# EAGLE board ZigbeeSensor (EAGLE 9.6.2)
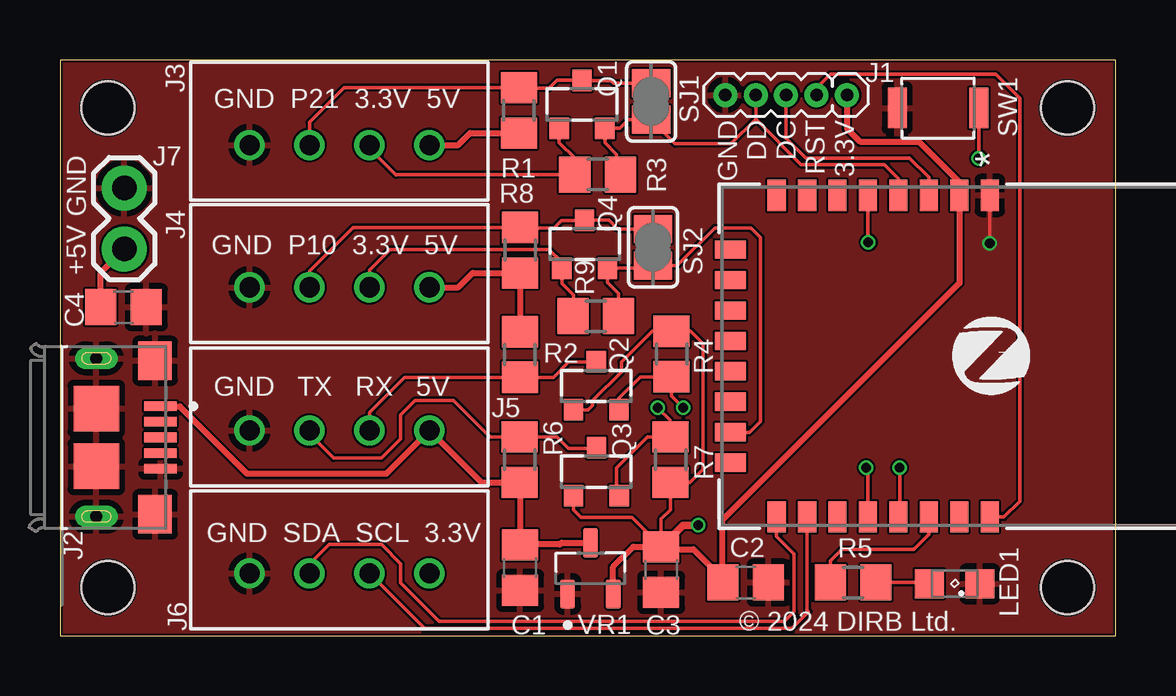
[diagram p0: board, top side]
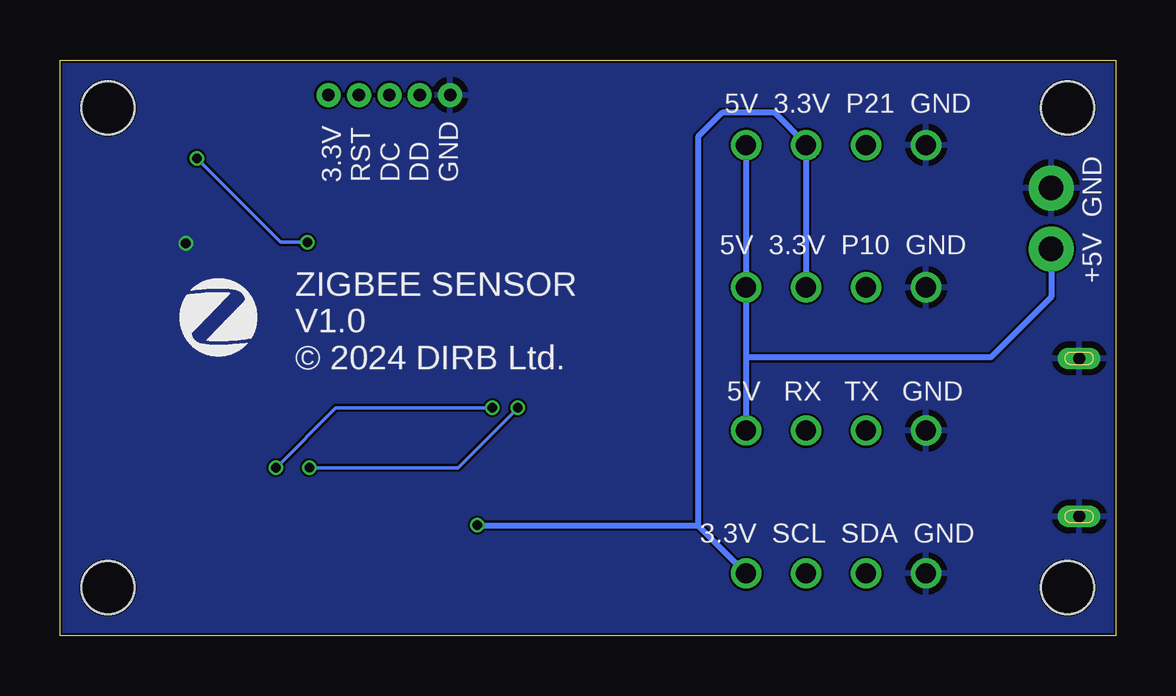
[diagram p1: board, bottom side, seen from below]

Size 44 x 24 mm. Coordinates in mm from the lower left corner, seen from the top.
Outline: 0,0 44,0 44,24 0,24 0,0
Copper layers (1*16): Top 0.035mm / dielectric 0.2mm / Bottom 0.035mm
Design rules "jlcpcb-2-layer": minimum track width 3.5mil, minimum drill 0.2mm, track to track 3.5mil, track to pad 5mil, pad to pad 5mil, via to via 5mil, smd to smd 0mil, copper to edge 0.1mm, drill to drill 5mil, minimum pad ring 4mil, minimum via ring 4mil, stop-mask expansion 3mil, vias tented up to drill 100mil, thermal gap 10mil
Holes 2.2 mm at 2,2 2,22 42,2 42,22

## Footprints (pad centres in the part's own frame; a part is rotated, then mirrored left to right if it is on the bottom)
C0805 = smd 1.3 x 1.5: 1 -0.95,0; 2 0.95,0
1X05_1.27MM = drill 0.508 pad 1: 1 0,0; 2 1.27,0; 3 2.54,0; 4 3.81,0; 5 5.08,0
AMPHENOL_10118193-0001LF = smd 0.4 x 1.35: 1 -1.3,2.675; 2 -0.65,2.675; 3 0,2.675; 4 0.65,2.675; 5 1.3,2.675 | smd 1.6 x 1.4: S1 -3.2,2.45; S2 3.2,2.45 | smd 1.9 x 1.9: S3 1.2,0; S4 -1.2,0 | drill 0.5 pad 0.9 long: S5 -3.3,0; S6 3.3,0
B4B-XH-A = drill 0.84: 1 0,0; 2 2.5,0; 3 5,0; 4 7.5,0
1X02 = drill 1.016 pad 1.88: 1 0,0; 2 2.54,0
SML0805 = smd 1.2 x 1.2: A 1.05,0; C -1.05,0
SOT23 = smd 0.8 x 0.9: 1 -0.95,-1; 2 0.95,-1; 3 0,1
R0805 = smd 1.3 x 1.5: 1 -0.95,0; 2 0.95,0
SJ = smd 1.168 x 1.6: 1 -0.762,0; 2 0.762,0
B3U-1000P = smd 0.8 x 1.7: 1 -1.7,0; 2 1.7,0
E18-MS1-PCB_BYT = smd 1.295 x 0.762: 1 -6.706,-0.35; 2 -6.706,-1.62; 3 -6.706,-2.89; 4 -6.706,-4.16; 5 -6.706,-5.43; 6 -6.706,-6.7; 7 -6.706,-7.97; 8 -6.706,-9.24; 17 6.706,-9.24; 18 6.706,-7.97; 19 6.706,-6.7; 20 6.706,-5.43; 21 6.706,-4.16; 22 6.706,-2.89; 23 6.706,-1.62; 24 6.706,-0.35 | smd 0.762 x 1.295: 9 -4.445,-11.163; 10 -3.175,-11.163; 11 -1.905,-11.163; 12 -0.635,-11.163; 13 0.635,-11.163; 14 1.905,-11.163; 15 3.175,-11.163; 16 4.445,-11.163
SOT95P237X112-3N = smd 1.22 x 0.62: 1 -1.065,0.95; 2 -1.065,-0.95; 3 1.065,0

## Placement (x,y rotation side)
C1  1u  [C0805]  19.18,2.83 270 top
C2  1u  [C0805]  28.58,2.21 0 top
C3  100n  [C0805]  25.06,2.75 270 top
C4  10u  [C0805]  2.65,13.69 0 top
J1  [1X05_1.27MM]  32.81,22.54 180 top
J2  10118193-0001LF  [AMPHENOL_10118193-0001LF]  1.52,8.26 270 top
J3  B4B-XH-A  [B4B-XH-A]  7.9,20.45 0 top
J4  B4B-XH-A  [B4B-XH-A]  7.9,14.52 0 top
J5  B4B-XH-A  [B4B-XH-A]  7.9,8.55 0 top
J6  B4B-XH-A  [B4B-XH-A]  7.9,2.59 0 top
J7  [1X02]  2.68,16.12 90 top
LED1  [SML0805]  37.29,2.16 180 top
Q1  BSS138  [SOT23]  21.76,22.15 0 top
Q2  BSS138  [SOT23]  22.35,10.41 0 top
Q3  BSS138  [SOT23]  22.36,6.83 0 top
Q4  BSS138  [SOT23]  21.87,16.32 0 top
R1  10K  [R0805]  19.13,21.9 270 top
R2  10K  [R0805]  19.17,11.72 90 top
R3  10K  [R0805]  22.41,19.22 180 top
R4  10K  [R0805]  25.49,11.74 90 top
R5  1K  [R0805]  33.06,2.21 180 top
R6  10K  [R0805]  19.16,7.33 270 top
R7  10K  [R0805]  25.45,7.33 270 top
R8  10K  [R0805]  19.18,16.07 270 top
R9  10K  [R0805]  22.33,13.32 180 top
SJ1  [SJ]  24.64,22.27 270 top
SJ2  [SJ]  24.72,16.19 270 top
SW1  B3U-1000P  [B3U-1000P]  36.6,22 0 top
U1  E18-MS1-PCB  [E18-MS1-PCB_BYT]  39.11,11.65 270 top
VR1  MCP1700T-3302E_TT  [SOT95P237X112-3N]  22.11,2.8 90 top

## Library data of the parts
C1-C4 = rcl; SPICEPREFIX: C
J1 J7 = SparkFun-Connectors
J2 = 10118193-0001LF; MANUFACTURER: Amphenol FCI; MAXIMUM_PACKAGE_HEIGHT: 2.55 mm; PARTREV: E; STANDARD: Manufacturer Recommendations
J3-J6 = Connector; CATEGORY: Header; DSECRIPTION: Connector Header Through Hole 4 position 0.098" (2.50mm); MANUFACTURER: JST Sales America Inc.; MPN: B4B-XH-A(LF)(SN); OPERATING_TEMPERATURE: -25 C to 85 C; PART_STATUS: ACTIVE; PITCH: 0.098" (2.50mm); ROHS_COMPLIANCE: ROHS3 Compliant; SERIES: XH; SUB_CATEGORY: Rectangular Connectors; TYPE: Header, Male Pin, Board to Cable/Wire, Through Hole
LED1 = led
Q1-Q4 = bss138_10; MF: Fairchild; MPN: BSS138; OC_FARNELL: 9845330; OC_NEWARK: 67R2009
R1-R9 = rcl; SPICEPREFIX: R
SJ1 SJ2 = jumper
SW1 = Switch; CREATED_BY: PCBLayout.com; DIGI_KEY_PART_NUMBER: SW1020CT-ND; MANUFACTURER: Omron Electronics Inc-EMC Div; MPN: B3U-1000P; PACKAGE: SPST-NO
U1 = 2024-03-18_07-21-07_Library; COPYRIGHT: Copyright (C) 2024 Ultra Librarian. All rights reserved.; MANUFACTURER_PART_NUMBER: E18-MS1-PCB; MFR_NAME: Chengdu Ebyte Elec Tech
VR1 = MCP1700T-3302E_TT; AVAILABILITY: In Stock; CHECK_PRICES: https://www.snapeda.com/parts/MCP1700T-3302E/TT/Microchip/view-part/?ref=eda; DESCRIPTION: Pwr Sply Func,Voltage Regulator,LDO,SOT-23,PD 369.6mW,VO 3.3V,Regline +/-0.75%/V | Microchip Technology Inc. MCP1700T-3302E/TT; MF: Microchip; MP: MCP1700T-3302E/TT; PACKAGE: SOT-23 Microchip; PRICE: None; PURCHASE-URL: https://www.snapeda.com/api/url_track_click_mouser/?unipart_id=8101&manufacturer=Microchip&part_name=MCP1700T-3302E/TT&search_term=None; SNAPEDA_LINK: https://www.snapeda.com/parts/MCP1700T-3302E/TT/Microchip/view-part/?ref=snap

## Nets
+3V3: C2.1 C3.1 J1.1 J3.3 J4.3 J6.4 Q1.1 Q2.1 Q3.1 Q4.1 R3.2 R4.2 R7.2 R9.2 U1.2 VR1.2
+5V: C1.1 C4.1 J2.1 J3.4 J4.4 J5.4 J7.1 R1.2 R2.2 R6.2 R8.2 VR1.3
DC: J1.3 U1.3
DD: J1.4 Q1.2 R3.1 SJ1.2 U1.4
GND: C1.2 C2.2 C3.2 C4.2 J1.5 J2.5 J2.S1 J2.S2 J2.S3 J2.S4 J2.S5 J2.S6 J3.1 J4.1 J5.1 J6.1 J7.2 LED1.C SW1.1 U1.1 VR1.1
N$1: J5.3 Q2.3 R2.1
N$2: R5.2 U1.22
N$3: J3.2 Q1.3 R1.1 SJ1.1
N$4: LED1.A R5.1
N$5: J4.2 Q4.3 R8.1 SJ2.1
N$6: SW1.2 U1.5
N$7: J5.2 Q3.3 R6.1
P10: Q4.2 R9.1 SJ2.2 U1.15
RESET: J1.2 U1.24
RX: Q2.2 R4.1 U1.21
SCL: J6.3 U1.18
SDA: J6.2 U1.17
TX: Q3.2 R7.1 U1.20

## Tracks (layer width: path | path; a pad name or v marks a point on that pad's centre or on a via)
+3V3  (via drill 0.4)
  Top 0.15: Q1.1 20.81,20.55 21.46,19.9 R3.2 | Q4.1 20.92,14.68 21.4,14.2 21.4,13.34 R9.2 | R4.2 25.8,12.69 26.29,12.69 26.8,12.18 26.8,6.93 26.25,6.38 R7.2 25.45,5.25 25.06,4.86 C3.1 23.84,4.92 21.71,4.92 21.41,5.23 Q3.1
  Top 0.152: R3.2 14.02,19.22 14,19.2 12.9,20.3 J3.3 | Q4.1 20.92,15.56 20.38,16.1 13.77,16.1 12.9,15.23 J4.3 | 25.8,12.69 24.69,12.69 23.4,11.4 23.4,11 22.2,9.8 22.2,9.6 22.01,9.41 Q2.1
  Top 0.254: VR1.2 23.06,2.86 23.9,3.7 C3.1 25.16,3.6 26.4,3.6 27.63,2.37 C2.1 27.6,2.24 27.6,4.8 37.49,14.69 U1.2 37.49,18.91 35.8,20.6 33.35,20.6 32.81,21.14 J1.1
  Top 0.305: C3.1 25.96,4.6 v26.6,4.6
  Bottom 0.254: J4.3 J3.3 12.9,20.5 14.2,21.8 16.4,21.8 17.4,20.8 17.4,4.6 | J6.4 17.4,4.6 | v26.6,4.6 17.4,4.6
+5V
  Top 0.254: J3.4 16.6,20.45 17.1,20.95 R1.2 | J4.4 16.6,14.52 17.2,15.12 R8.2 R2.2 | VR1.3 20.91,3.87 20.84,3.8 19.2,3.8 C1.1 19.18,6.36 R6.2 17.57,6.38 J5.4 13.6,6.75 7.8,6.75 4.99,9.56 J2.1 | C4.1 1.7,15.14 J7.1
  Bottom 0.254: J7.1 2.68,14.12 5.2,11.6 15.35,11.6 15.4,11.55 J5.4 J4.4 J3.4
DC
  Top 0.15: J1.3 30.27,20.73 31.09,19.91 35.41,19.91 36.22,19.1 U1.3
DD
  Top 0.15: R3.1 23.2,19.38 23.2,20.06 22.71,20.55 Q1.2 23.35,21.15 23.71,21.51 SJ1.2 25.64,20.51 27.97,20.51 29,21.54 J1.4 29,21.53 30.89,19.64 34.36,19.64 34.95,19.05 U1.4
GND  (via drill 0.4)
  Top 0.15: U1.1 38.76,16.44 38.8,16.4 38.8,16.39 v38.76,16.35
  pour Top: 0,0 44,0 44,24 0,24
  pour Bottom: 0,0 44,0 44,24 0,24
N$1
  Top 0.152: J5.3 12.9,9.3 14.37,10.77 R2.1 20.57,10.77 21.2,11.4 Q2.3
N$2
  Top 0.152: R5.2 32.11,3.11 32.6,3.6 35.6,3.6 36.22,4.22 U1.22
N$3
  Top 0.15: SJ1.1 23.07,23.03 22.96,23.14 21.77,23.14 Q1.3 20.73,23.15 20.39,22.82 19.16,22.82 R1.1 11.85,22.85 10.4,21.4 J3.2
N$4
  Top 0.152: R5.1 36.19,2.21 LED1.A
N$5
  Top 0.15: Q4.3 22.88,17.32 23.25,16.95 SJ2.1 | R8.1 12.22,17.02 10.4,15.2 J4.2
  Top 0.152: Q4.3 21.86,17.31 20.91,17.31 20.6,17 19.2,17 R8.1
N$6  (via drill 0.4)
  Top 0.15: SW1.2 38.3,20.1 38.4,20 v38.3,19.9 | v33.69,16.4 33.68,16.41 U1.5
  Bottom 0.15: v38.3,19.9 34.8,16.4 v33.69,16.4
N$7
  Top 0.152: Q3.3 22.33,7.8 21.2,7.8 20.73,8.28 R6.1 17.92,8.28 16.4,9.8 14.8,9.8 14.2,9.2 14.2,8.2 13.4,7.4 11.4,7.4 10.4,8.4 J5.2
P10
  Top 0.15: R9.1 23.28,14.26 22.82,14.72 Q4.2 24.61,15.32 SJ2.2 25.72,15.43 27.29,17 28.8,17 29.2,16.6 29.2,8.93 28.75,8.47 U1.15
RESET
  Top 0.15: J1.2 31.6,22.6 31.6,22.89 32.11,23.4 39,23.4 40,22.4 40,5.6 39.34,4.94 U1.24
RX  (via drill 0.4)
  Top 0.152: Q2.2 23.3,9.9 24.19,10.79 R4.1 25.49,9.99 v25.98,9.5 | v35,7 35,4.99 U1.21
  Bottom 0.152: v25.98,9.5 32.5,9.5 v35,7
SCL
  Top 0.152: U1.18 31.14,1.06 31.2,1 30.5,0.3 15.19,0.3 J6.3
SDA
  Top 0.152: J6.2 10.4,2.99 11.21,3.8 13.4,3.8 14.2,3 14.2,2.2 15.8,0.6 30.2,0.6 30.6,1 30.6,3.4 29.87,4.13 U1.17
TX  (via drill 0.4)
  Top 0.152: Q3.2 23.2,5.94 23.2,7 24.48,8.28 R7.1 25.43,8.3 25.43,8.98 v24.91,9.5 | v33.6,7 33.68,6.92 U1.20
  Bottom 0.152: v24.91,9.5 27.41,7 v33.6,7

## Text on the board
tNames: GND P21 3.3V 5V | GND / DD / DC / RST / 3.3V | GND | GND P10 3.3V 5V | +5V | GND TX RX 5V | GND SDA SCL 3.3V | © 2024 DIRB Ltd.
bNames: 5V 3.3V P21 GND | GND | 3.3V / RST / DC / DD / GND | +5V | 5V 3.3V P10 GND | ZIGBEE SENSOR / V1.0 / © 2024 DIRB Ltd. | 5V RX TX GND | 3.3V SCL SDA GND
